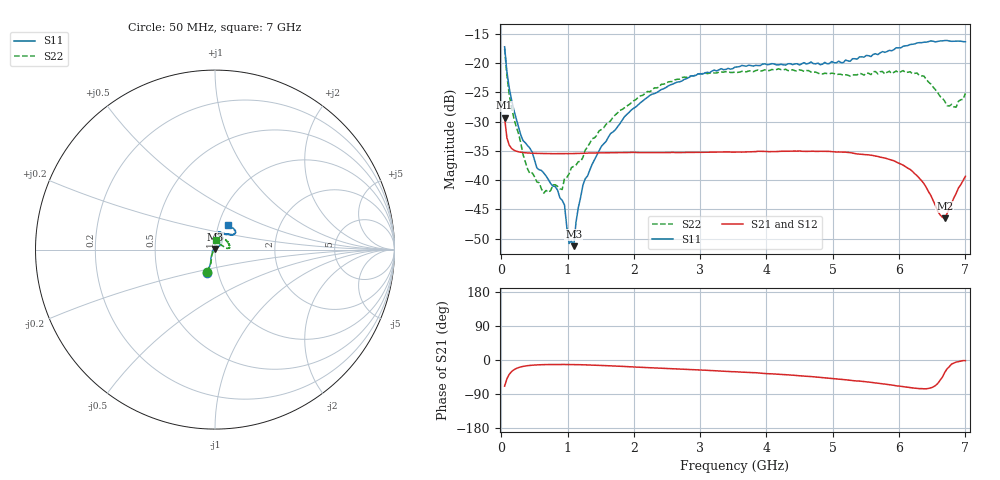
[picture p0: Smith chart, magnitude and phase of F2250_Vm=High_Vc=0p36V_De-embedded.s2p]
! Integrated Device Technology
! Corporate Headquarters
! 6024 Silver Creek Valley Road
! San Jose, CA 95138  USA
! Phone:  1-408-284-8200
! Toll Free:  1-800-223-1366
! Webpage:  http://www.idt.com/
! Timing and RF Division
! 515 Groton Road, Suite 102
! Westford, MA 01886-6024
! Device:  F2250
! Description: Voltage Variable RF Attenuator
! Frequency:  50.0 -  6000.00 MHz
! Package:  3x3 mm Thin QFN Plastic Package: 16 pin
! Ports:  2 RF, 3 DC
!  Pin  1  = GND
!  Pin  2  = NC
!  Pin  3  = RF1  = Port 1
!  Pin  4  = NC
!  Pin  5  = GND
!  Pin  6  = GND
!  Pin  7  = GND
!  Pin  8  = GND
!  Pin  9  = NC
!  Pin 10  = RF2  = Port 2
!  Pin 11  = NC
!  Pin 12  = GND
!  Pin 13  = GND
!  Pin 14  = VCNTRL
!  Pin 15  = VDD
!  Pin 16  = VMODE
! Vcntrl:  0.360 Volts
! Vmode:  +3.300 Volts
! Vdd:  +3.30  Volts
! Current:  1.260 mA
! Data:  The device was measured on a the F2250 evaluation board which has
!  individual transmission lines to the RF pins.  Data was collected
!  using a calibrated network analyzer.  The evaluation board was
!  de-embedded using a TRL calibration technique.
!  The reference plane is the edge of the package pin.
! Misc:  SN 10
!  Action Tracker AT0258
! Date Measured:  2014-11-26
! Date:  2015-10-15  MJV
! Note:
!  Integrated Device Technology supplies this data as a sample of measured
!  data at the package pin for this product.  Your particular data for this
!  product may vary.
!  Data was taken at 25 degrees C.
!  Integrated Device Technology reserves the right to change this data at anytime.
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# GHz S dB R 50
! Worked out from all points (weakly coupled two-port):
!   201 points, 50 MHz to 7 GHz, reference 50 ohm
!   highest |S21| = -29.34 dB at 50 MHz (marker M1); lowest = -46.5 dB at 6.687 GHz (marker M2)
!   lowest |S11| = -51.3 dB at 1.093 GHz (marker M3), VSWR 1.01, Z = 50 + j0.272 ohm
!   |S11| at or under -10 dB: start of sweep to end of sweep
!   |S22| runs from -42.2 to -17.5 dB; largest |S21 - S12| = 5.4e-05
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0.05  -17.18 -108.5  -29.34 -69.0  -29.34 -69.0  -17.54 -109.8
0.08475  -21.47 -107.4  -32.77 -49.6  -32.77 -49.6  -22.11 -107.0
0.189  -27.99 -119.9  -34.86 -25.9  -34.86 -25.9  -29.36 -119.7
0.328  -33.24 -134.0  -35.28 -16.9  -35.28 -16.9  -35.63 -133.6
0.43225  -34.55 -145.3  -35.38 -14.2  -35.38 -14.2  -38.89 -162.5
0.5365  -37.91 -154.7  -35.43 -12.9  -35.42 -12.9  -40.31 -177.4
0.64075  -38.78 -162.7  -35.45 -12.2  -35.45 -12.2  -42.22 155.6
0.91875  -43.46 156.1  -35.48 -11.8  -35.48 -11.8  -41.60 112.1
0.9535  -44.26 170.7  -35.47 -11.9  -35.47 -11.9  -39.70 110.6
1.023  -50.85 140.8  -35.46 -12.0  -35.46 -11.9  -38.91 92.6
1.0925  -51.30 89.4  -35.44 -12.1  -35.45 -12.1  -37.63 84.0
1.12725  -47.17 61.1  -35.44 -12.2  -35.44 -12.2  -37.41 77.0
1.2315  -40.84 40.6  -35.40 -12.6  -35.40 -12.6  -36.10 63.8
1.6485  -32.03 41.2  -35.32 -15.3  -35.32 -15.4  -29.84 53.5
2.37825  -24.76 46.7  -35.28 -21.3  -35.28 -21.3  -24.07 50.6
3.525  -20.65 71.7  -35.21 -30.9  -35.21 -31.0  -21.52 71.3
4.7065  -20.06 72.0  -35.05 -44.3  -35.05 -44.3  -21.53 69.3
5.85325  -17.79 40.5  -36.47 -65.2  -36.47 -65.3  -21.37 21.8
6.3745  -16.40 40.9  -40.59 -76.0  -40.62 -76.1  -22.19 5.6
6.68725  -16.11 47.9  -46.52 -33.5  -46.51 -32.9  -26.47 27.2
6.861  -16.21 54.5  -42.27 -5.5  -42.25 -5.6  -27.50 57.7
7  -16.32 62.4  -39.34 -1.6  -39.31 -1.7  -25.15 85.0
